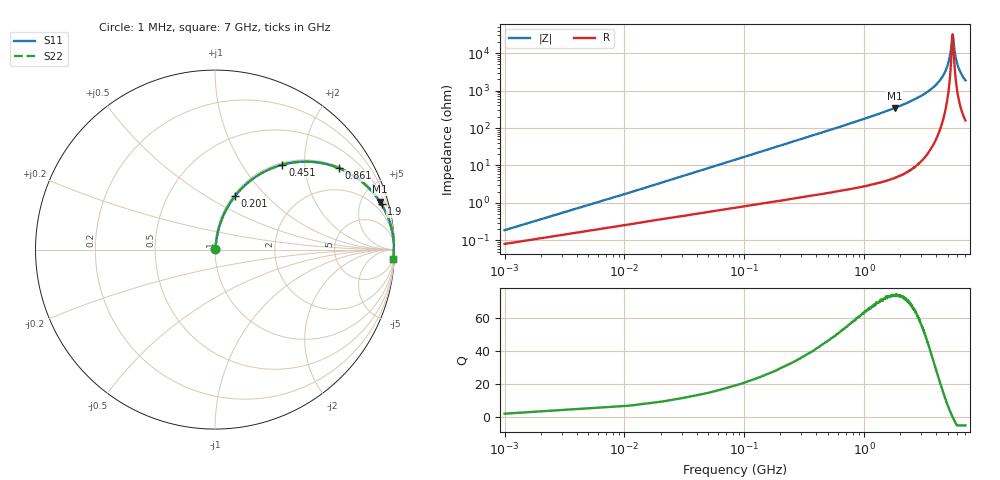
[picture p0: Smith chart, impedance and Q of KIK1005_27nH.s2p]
!version-3
!date-01.2023
!Series
# MHz S RI R 50
!Freq ReS11 ImS11 ReS21 ImS21 ReS12 ImS12 ReS22 ImS22
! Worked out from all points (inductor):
!   701 points, 1 MHz to 7 GHz, reference 50 ohm
!   read as one part in series: L = 27 nH near 31 MHz
!   highest Q = 73.8 at 1.8 GHz (marker M1), where L = 30.3 nH
!   self-resonance near 5.48 GHz
!   S11 on the Smith chart (normalised r, x): 1 MHz: 1.00, +0.00; 201 MHz: 1.02, +0.68; 451 MHz: 1.03, +1.54; 861 MHz: 1.05, +3.00; 1.9 GHz: 1.10, +7.33; 7 GHz: 4, -37
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1  0.000815 0.00169  0.9992 -0.00169  0.9992 -0.00169  0.000815 0.00169
41  0.00992 0.0685  0.9901 -0.0685  0.9901 -0.0685  0.00992 0.0685
61  0.0167 0.1011  0.9833 -0.1011  0.9833 -0.1011  0.0167 0.1011
121  0.0483 0.1937  0.9517 -0.1937  0.9517 -0.1937  0.0483 0.1937
201  0.1125 0.2996  0.8875 -0.2996  0.8875 -0.2996  0.1125 0.2996
451  0.3753 0.473  0.6247 -0.473  0.6247 -0.473  0.3753 0.473
861  0.6888 0.4547  0.3112 -0.4547  0.3112 -0.4547  0.6888 0.4547
1170  0.8089 0.3858  0.1911 -0.3858  0.1911 -0.3858  0.8089 0.3858
1800  0.9184 0.267  0.0816 -0.267  0.0816 -0.267  0.9184 0.267
1900  0.9278 0.2521  0.0722 -0.2521  0.0722 -0.2521  0.9278 0.2521
2340  0.9568 0.1964  0.0432 -0.1964  0.0432 -0.1964  0.9568 0.1964
3510  0.988 0.0976  0.012 -0.0976  0.012 -0.0976  0.988 0.0976
4670  0.9961 0.0343  0.00386 -0.0343  0.00386 -0.0343  0.9961 0.0343
4940  0.9967 0.0222  0.00332 -0.0222  0.00332 -0.0222  0.9967 0.0222
5150  0.9969 0.0133  0.00312 -0.0133  0.00312 -0.0133  0.9969 0.0133
5280  0.9969 0.00796  0.00309 -0.00796  0.00309 -0.00796  0.9969 0.00796
5470  0.9968 0.000405  0.00316 -0.000405  0.00316 -0.000405  0.9968 0.000405
5520  0.9968 -0.00154  0.0032 0.00154  0.0032 0.00154  0.9968 -0.00154
5700  0.9966 -0.00839  0.0034 0.00839  0.0034 0.00839  0.9966 -0.00839
5840  0.9964 -0.0136  0.00362 0.0136  0.00362 0.0136  0.9964 -0.0136
6290  0.9953 -0.0295  0.00469 0.0295  0.00469 0.0295  0.9953 -0.0295
7000  0.9927 -0.0524  0.00728 0.0524  0.00728 0.0524  0.9927 -0.0524
